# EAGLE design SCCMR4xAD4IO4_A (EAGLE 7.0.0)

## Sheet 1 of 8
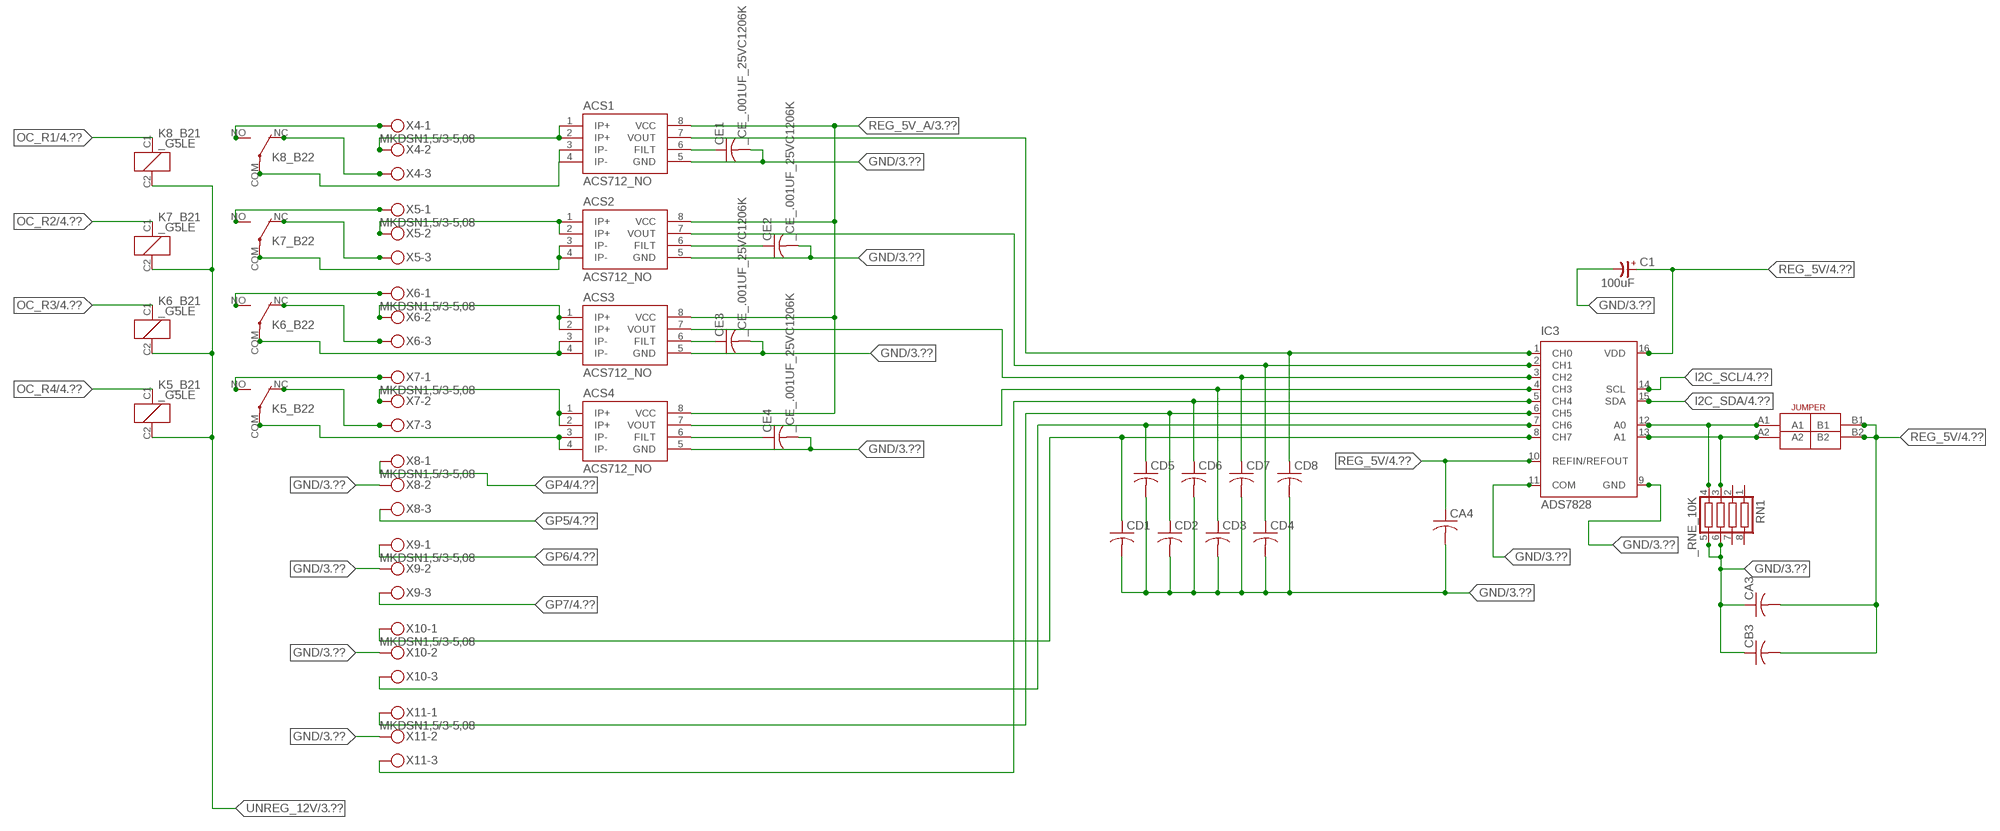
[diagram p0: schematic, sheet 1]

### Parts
ACS1  ACS712_NO  [_MA_DUAL_N-FET]
ACS2  ACS712_NO  [_MA_DUAL_N-FET]
ACS3  ACS712_NO  [_MA_DUAL_N-FET]
ACS4  ACS712_NO  [_MA_DUAL_N-FET]
C1  100uF  CP-E-025X060  [E-025X060]
CA3  CC1206KRX7R9BB104C1206K  [CC1206KRX7R9BB104]
CA4  CC1206KRX7R9BB104C1206K  [CC1206KRX7R9BB104]
CB3  TMK316F106ZL-TC1206K  [TMK316F106ZL-T]
CD1  _CD_10NF_50VC1206K  [_CD_10NF_50V]
CD2  _CD_10NF_50VC1206K  [_CD_10NF_50V]
CD3  _CD_10NF_50VC1206K  [_CD_10NF_50V]
CD4  _CD_10NF_50VC1206K  [_CD_10NF_50V]
CD5  _CD_10NF_50VC1206K  [_CD_10NF_50V]
CD6  _CD_10NF_50VC1206K  [_CD_10NF_50V]
CD7  _CD_10NF_50VC1206K  [_CD_10NF_50V]
CD8  _CD_10NF_50VC1206K  [_CD_10NF_50V]
CE1  _CE_.001UF_25VC1206K  [CE]
CE2  _CE_.001UF_25VC1206K  [CE]
CE3  _CE_.001UF_25VC1206K  [CE]
CE4  _CE_.001UF_25VC1206K  [CE]
IC3  ADS7828  [TSSOP16-PW]
K5_B2  _G5LE  [G5LE]
K6_B2  _G5LE  [G5LE]
K7_B2  _G5LE  [G5LE]
K8_B2  _G5LE  [G5LE]
RN1  _RNE_10K  [RNE]
U$4  JUMPER_2X2  [JUMPER_2X2]
X4  MKDSN1,5/3-5,08  [MKDSN1,5/3-5,08]
X5  MKDSN1,5/3-5,08  [MKDSN1,5/3-5,08]
X6  MKDSN1,5/3-5,08  [MKDSN1,5/3-5,08]
X7  MKDSN1,5/3-5,08  [MKDSN1,5/3-5,08]
X8  MKDSN1,5/3-5,08  [MKDSN1,5/3-5,08]
X9  MKDSN1,5/3-5,08  [MKDSN1,5/3-5,08]
X10  MKDSN1,5/3-5,08  [MKDSN1,5/3-5,08]
X11  MKDSN1,5/3-5,08  [MKDSN1,5/3-5,08]

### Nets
GND: ACS1.5(GND) ACS2.5(GND) ACS3.5(GND) ACS4.5(GND) C1.- CA3.1 CA4.2 CB3.1 CD1.2 CD2.2 CD3.2 CD4.2 CD5.2 CD6.2 CD7.2 CD8.2 CE1.2 CE2.2 CE3.2 CE4.2 IC3.9(GND) IC3.11(COM) RN1.5 RN1.6 X8.2 X9.2 X10.2 X11.2 ; also sheet 3,4,6,8
GP4: X8.1 ; also sheet 4
GP5: X8.3 ; also sheet 4
GP6: X9.1 ; also sheet 4
GP7: X9.3 ; also sheet 4
I2C_SCL: IC3.14(SCL) ; also sheet 4,6
I2C_SDA: IC3.15(SDA) ; also sheet 4,6
N$7: ACS1.1(IP+) ACS1.2(IP+) X4.2
N$8: CD5.1 IC3.7(CH6) X10.3
N$9: ACS1.7(VOUT) CD8.1 IC3.1(CH0)
N$10: ACS2.7(VOUT) CD4.1 IC3.2(CH1)
N$11: ACS3.7(VOUT) CD7.1 IC3.3(CH2)
N$12: ACS4.7(VOUT) CD3.1 IC3.4(CH3)
N$13: ACS2.1(IP+) ACS2.2(IP+) X5.2
N$17: IC3.12(A0) RN1.4 U$4.A1
N$18: IC3.13(A1) RN1.3 U$4.A2
N$20: CD2.1 IC3.6(CH5) X11.1
N$21: ACS4.1(IP+) ACS4.2(IP+) X7.2
N$22: ACS4.3(IP-) ACS4.4(IP-) K5_B2.COM(2:COM)
N$24: CD1.1 IC3.8(CH7) X10.1
N$25: CD6.1 IC3.5(CH4) X11.3
N$33: ACS1.6(FILT) CE1.1
N$34: ACS2.6(FILT) CE2.1
N$35: ACS3.6(FILT) CE3.1
N$36: ACS4.6(FILT) CE4.1
N$42: ACS1.3(IP-) ACS1.4(IP-) K8_B2.COM(2:COM)
N$43: K8_B2.NC(2:NC) X4.3
N$44: K8_B2.NO(2:NO) X4.1
N$45: K7_B2.NO(2:NO) X5.1
N$46: K6_B2.NO(2:NO) X6.1
N$137: K7_B2.NC(2:NC) X5.3
N$138: ACS2.3(IP-) ACS2.4(IP-) K7_B2.COM(2:COM)
N$139: K6_B2.NC(2:NC) X6.3
N$140: ACS3.3(IP-) ACS3.4(IP-) K6_B2.COM(2:COM)
N$141: K5_B2.NC(2:NC) X7.3
N$143: K5_B2.NO(2:NO) X7.1
N$166: ACS3.1(IP+) ACS3.2(IP+) X6.2
OC_R1: K8_B2.C1(1:C1) ; also sheet 4
OC_R2: K7_B2.C1(1:C1) ; also sheet 4
OC_R3: K6_B2.C1(1:C1) ; also sheet 4
OC_R4: K5_B2.C1(1:C1) ; also sheet 4
REG_5V: C1.+ CA3.2 CA4.1 CB3.2 IC3.10(REFIN/REFOUT) IC3.16(VDD) U$4.B1 U$4.B2 ; also sheet 4,6,8
REG_5V_A: ACS1.8(VCC) ACS2.8(VCC) ACS3.8(VCC) ACS4.8(VCC) ; also sheet 3
UNREG_12V: K5_B2.C2(1:C2) K6_B2.C2(1:C2) K7_B2.C2(1:C2) K8_B2.C2(1:C2) ; also sheet 3,4,6
Unconnected: RN1.1 RN1.2 RN1.7 RN1.8

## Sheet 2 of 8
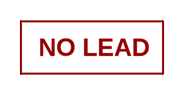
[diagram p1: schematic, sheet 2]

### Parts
U$16  NOPB_LOGO_SYM  [NOPB_LOGO_SYM]

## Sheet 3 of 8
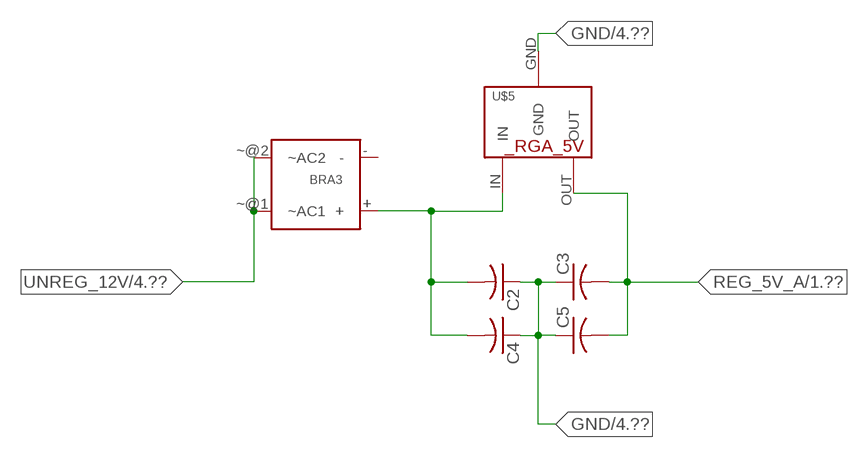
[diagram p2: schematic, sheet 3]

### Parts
BRA3  MB2S_  [MB2S]
C2  _CA_.10UF_50VC1206K  [_CA_.1UF_50V]
C3  _CA_.10UF_50VC1206K  [_CA_.1UF_50V]
C4  _CB_10UF_25VC1206K  [_CB_10UF_25V]
C5  _CB_10UF_25VC1206K  [_CB_10UF_25V]
U$5  _RGA_5V  [_RGA_5V]

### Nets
GND: C2.1 C3.1 C4.1 C5.1 U$5.GND ; also sheet 1,4,6,8
N$31: BRA3.+ C2.2 C4.2 U$5.IN
REG_5V_A: C3.2 C5.2 U$5.OUT ; also sheet 1
UNREG_12V: BRA3.~@1(~AC1) BRA3.~@2(~AC2) ; also sheet 1,4,6
Unconnected: BRA3.-

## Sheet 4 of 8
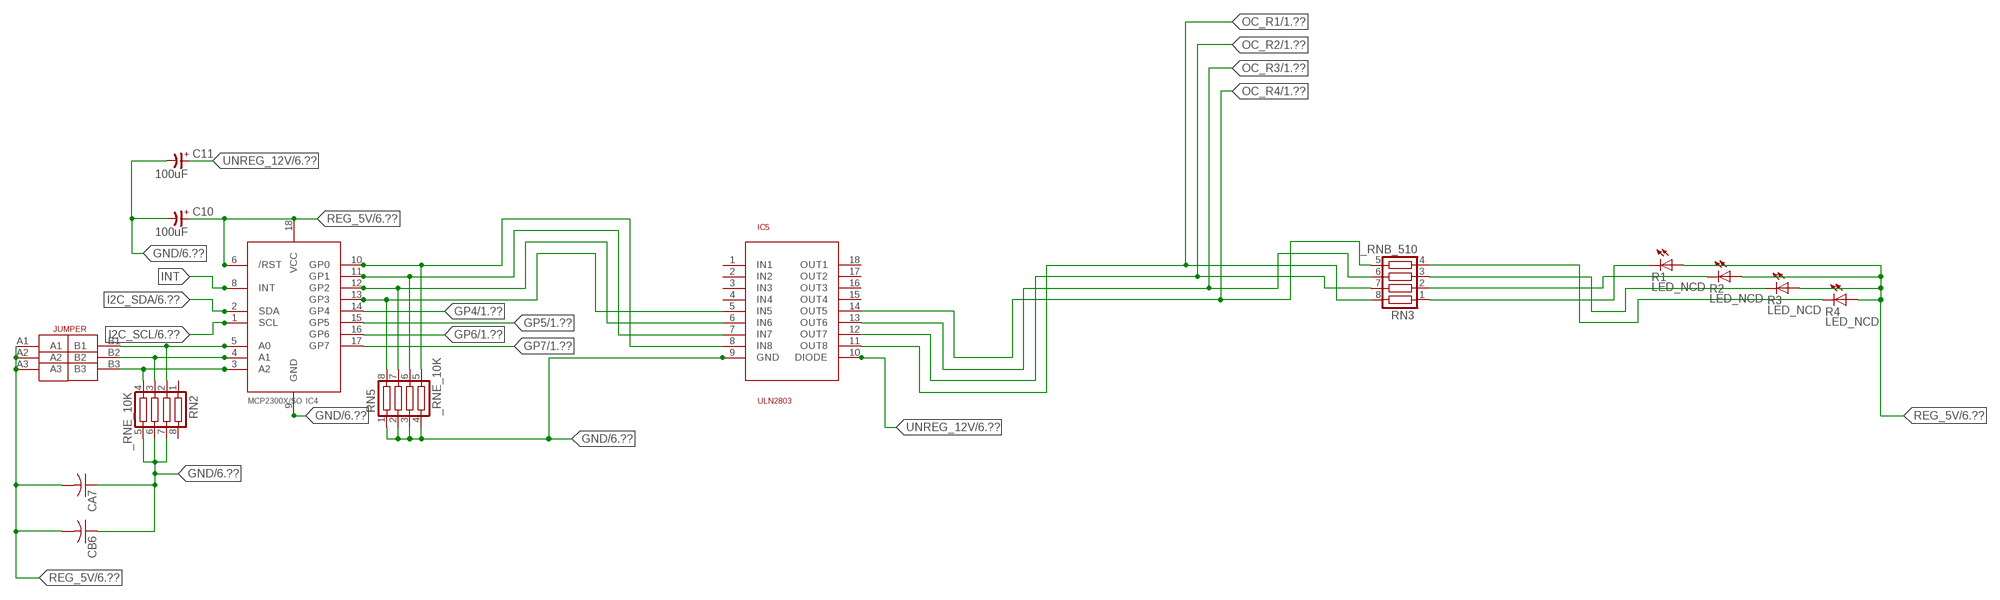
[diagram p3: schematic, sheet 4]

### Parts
C10  100uF  CP-E-025X060  [E-025X060]
C11  100uF  CP-E-025X060  [E-025X060]
CA7  CC1206KRX7R9BB104C1206K  [CC1206KRX7R9BB104]
CB6  TMK316F106ZL-TC1206K  [TMK316F106ZL-T]
IC4  MCP2300X/SO  [SO18W]
IC5  ULN2803  [SO18L]
R1  LED_NCD  [CHIPLED_0603]
R2  LED_NCD  [CHIPLED_0603]
R3  LED_NCD  [CHIPLED_0603]
R4  LED_NCD  [CHIPLED_0603]
RN2  _RNE_10K  [RNE]
RN3  _RNB_510  [RNB]
RN5  _RNE_10K  [RNE]
U$18  JUMPER_3X2  [JUMPER_3X2]

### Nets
GND: C10.- C11.- CA7.1 CB6.1 IC4.9(GND) IC5.9(GND) RN2.5 RN2.6 RN2.7 RN5.1 RN5.2 RN5.3 RN5.4 ; also sheet 1,3,6,8
GP4: IC4.14(GP4) ; also sheet 1
GP5: IC4.15(GP5) ; also sheet 1
GP6: IC4.16(GP6) ; also sheet 1
GP7: IC4.17(GP7) ; also sheet 1
I2C_SCL: IC4.1(SCL) ; also sheet 1,6
I2C_SDA: IC4.2(SDA) ; also sheet 1,6
INT: IC4.8(INT)
N$47: IC4.5(A0) RN2.2 U$18.B1
N$48: IC4.4(A1) RN2.3 U$18.B2
N$49: IC4.3(A2) RN2.4 U$18.B3
N$50: IC4.12(GP2) IC5.6(IN6) RN5.7
N$51: IC4.11(GP1) IC5.7(IN7) RN5.6
N$52: IC4.10(GP0) IC5.8(IN8) RN5.5
N$53: R1.C RN3.1
N$54: R2.C RN3.2
N$55: R3.C RN3.3
N$56: R4.C RN3.4
N$89: IC4.13(GP3) IC5.5(IN5) RN5.8
OC_R1: IC5.11(OUT8) RN3.8 ; also sheet 1
OC_R2: IC5.12(OUT7) RN3.7 ; also sheet 1
OC_R3: IC5.13(OUT6) RN3.6 ; also sheet 1
OC_R4: IC5.14(OUT5) RN3.5 ; also sheet 1
REG_5V: C10.+ CA7.2 CB6.2 IC4.6(/RST) IC4.18(VCC) R1.A R2.A R3.A R4.A U$18.A1 U$18.A2 U$18.A3 ; also sheet 1,6,8
UNREG_12V: C11.+ IC5.10(DIODE) ; also sheet 1,3,6
Unconnected: IC5.1(IN1) IC5.2(IN2) IC5.3(IN3) IC5.4(IN4) IC5.15(OUT4) IC5.16(OUT3) IC5.17(OUT2) IC5.18(OUT1) RN2.1 RN2.8

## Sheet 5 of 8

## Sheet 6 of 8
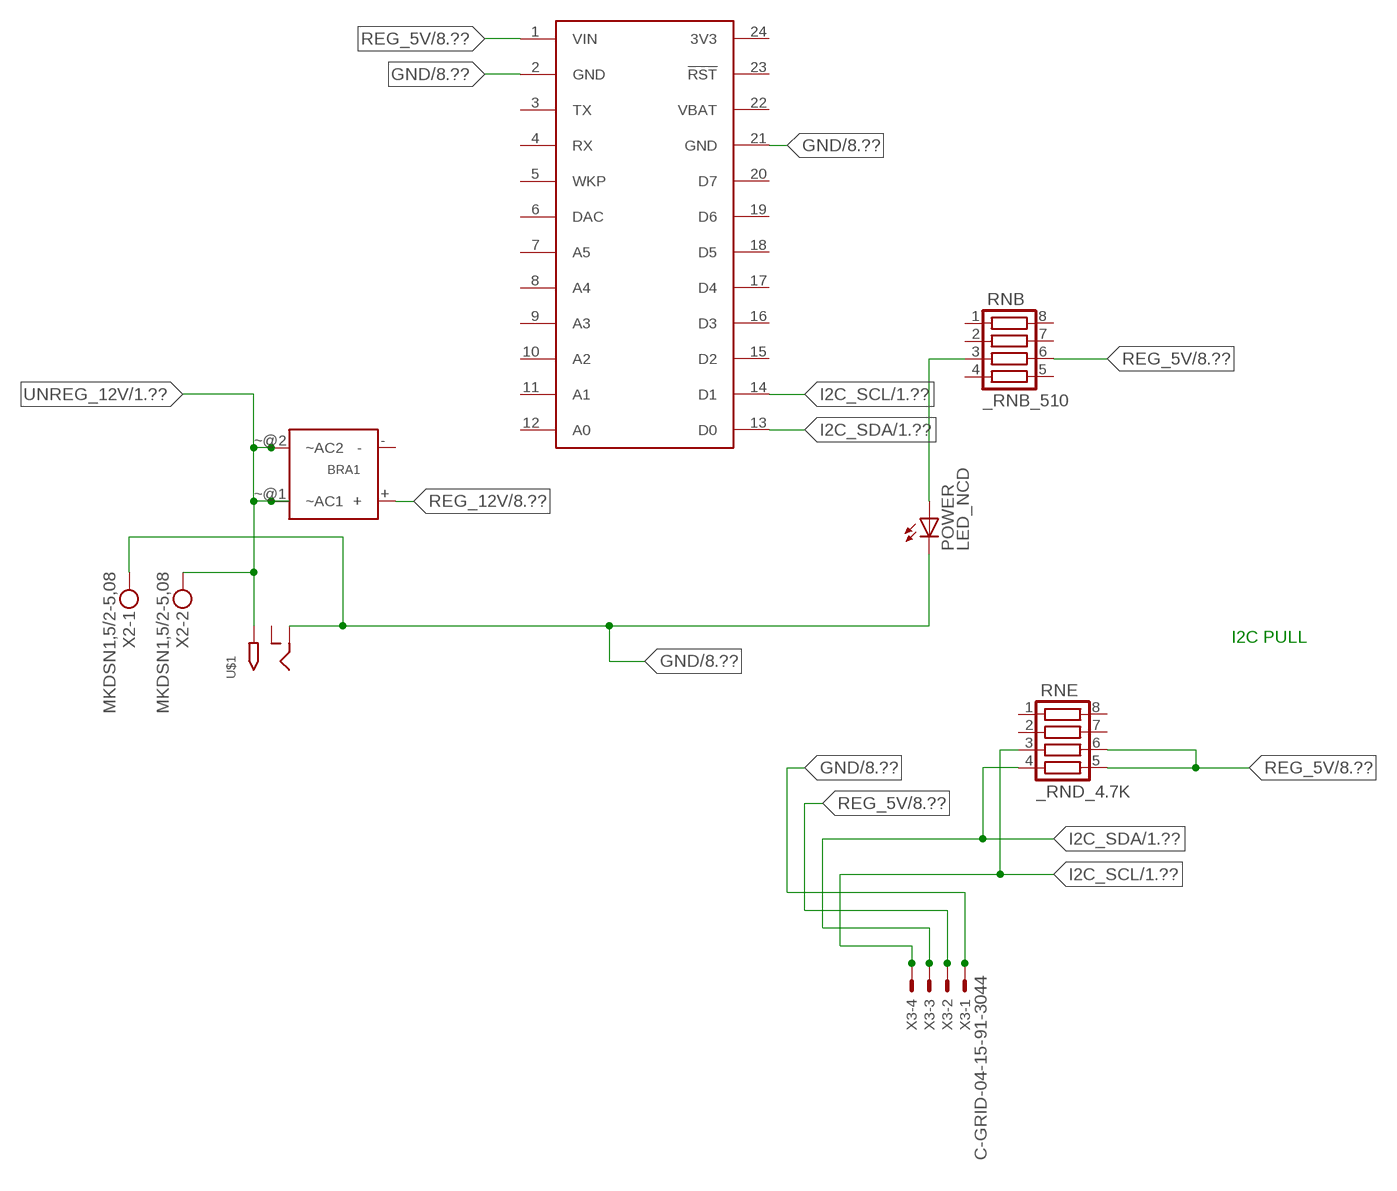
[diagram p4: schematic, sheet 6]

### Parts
BRA1  MB2S_  [MB2S]
POWER  LED_NCD  [CHIPLED_0603]
RNB  _RNB_510  [RNB]
RNE  _RND_4.7K  [RND]
S1  SPARK_CORECORE  [SPARK_CORE]
U$1  2.1MMJACK  [PJ-102A]
X2  MKDSN1,5/2-5,08  [MKDSN1,5/2-5,08]
X3  C-GRID-04-15-91-3044  [15-91-04]

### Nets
GND: POWER.C S1.2(GND) S1.21(GND) U$1.RING X2.1 X3.1 ; also sheet 1,3,4,8
I2C_SCL: RNE.3 S1.14(D1) X3.4 ; also sheet 1,4
I2C_SDA: RNE.4 S1.13(D0) X3.3 ; also sheet 1,4
N$2: POWER.A RNB.3
REG_5V: RNB.6 RNE.5 RNE.6 S1.1(VIN) X3.2 ; also sheet 1,4,8
REG_12V: BRA1.+ ; also sheet 8
UNREG_12V: BRA1.~@1(~AC1) BRA1.~@2(~AC2) U$1.TIP X2.2 ; also sheet 1,3,4
Unconnected: BRA1.- RNB.1 RNB.2 RNB.4 RNB.5 RNB.7 RNB.8 RNE.1 RNE.2 RNE.7 RNE.8 S1.3(TX) S1.4(RX) S1.5(WKP) S1.6(DAC) S1.7(A5) S1.8(A4) S1.9(A3) S1.10(A2) S1.11(A1) S1.12(A0) S1.15(D2) S1.16(D3) S1.17(D4) S1.18(D5) S1.19(D6) S1.20(D7) S1.23(!RST) U$1.RING_SW

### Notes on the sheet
- I2C PULL

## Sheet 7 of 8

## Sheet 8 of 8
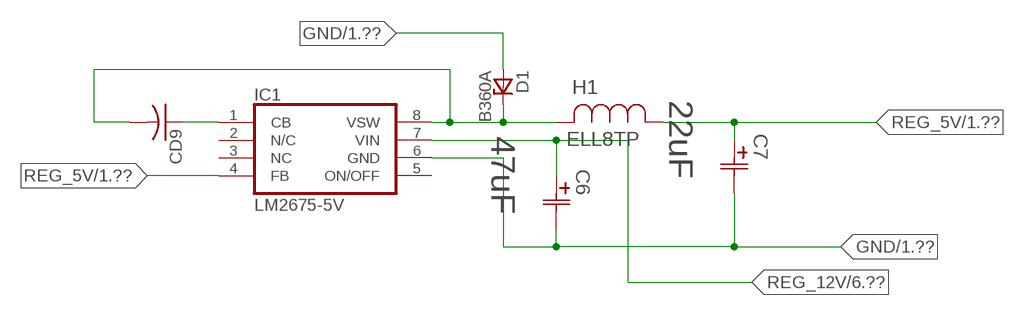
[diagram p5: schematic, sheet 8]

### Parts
C6  47uF  490-5463-6-NDCAP  [C2917(7343)-Y]
C7  22uF  490-5463-6-NDCAP  [C2917(7343)-Y]
CD9  _CD_10NF_50VC1206K  [_CD_10NF_50V]
D1  B360A  [DO214AC_ZENER]
H1  ELL8TP  [IND_ELL8TP]
IC1  LM2675-5V  LM2675  [SO-8]

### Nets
GND: C6.2(C2) C7.2(C2) D1.A IC1.6(GND) ; also sheet 1,3,4,6
N$1: CD9.2 D1.C H1.2 IC1.8(VSW)
N$6: CD9.1 IC1.1(CB)
REG_5V: C7.1(C1) H1.1 IC1.4(FB) ; also sheet 1,4,6
REG_12V: C6.1(C1) IC1.7(VIN) ; also sheet 6
Unconnected: IC1.2(N/C) IC1.5(ON/OFF)

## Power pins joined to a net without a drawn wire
3V3: S1.24(3V3)
NC: IC1.3(NC)
VBAT: S1.22(VBAT)

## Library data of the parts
ACS1-ACS4 = NCD_ULTIMATE_LIBRARY:ACS712_NO: Semiconductor Sensor Current Hall-effect-based isolated linear current sensor Digikey 620-1190-2-ND/ACS712ELCTR-20A-T
BRA1 BRA3 = NCD_ULTIMATE_LIBRARY:MB2S: Bridge Rectifier BRA MB2S 200V 500ma Digikey MB2S-TPMSTR-ND/MB2S-TP
C1 C10 C11 = NCD_ULTIMATE_LIBRARY:CP-: Capacitors All Kinds POLARIZED CAP
C2 C3 = NCD_ULTIMATE_LIBRARY:_CA_.10UF_50V: Capacitor .1uF SMT
C4 C5 = NCD_ULTIMATE_LIBRARY:_CB_10UF_25V: Capacitor 10uF SMT
C6 C7 = NCD_ULTIMATE_bhaskar:490-5463-6-ND: NCD CAP
CA3 CA4 CA7 = NCD_ULTIMATE_LIBRARY:CC1206KRX7R9BB104: Capacitor CA .1uF 50V SMT C1206K CC1206KRX7R9BB104
CB3 CB6 = NCD_ULTIMATE_LIBRARY:TMK316F106ZL-T: Capacitor CB 10uF SMT 1206 TMK316F106ZL-T
CD1-CD9 = NCD_ULTIMATE_LIBRARY:_CD_10NF_50V: Capacitor 10nF SMT
CE1-CE4 = NCD_ULTIMATE_LIBRARY:_CE_.001UF_25V: Capacitor .001uF SMT
D1 = NCD_ULTIMATE_bhaskar:B360A: NCD DIODE B350A/B360A
H1 = NCD_ULTIMATE_bhaskar:ELL8TP: NCD coil
IC1 = NCD_ULTIMATE_bhaskar:LM2675: LM2675 NCD http://www.ti.com/lit/ds/symlink/lm2675.pdf
IC3 = NCD_ULTIMATE_LIBRARY:ADS7828: Semiconductor ADC I2C 12-Bit, 8-Channel Sampling ANALOG-TO-DIGITAL CONVERTER Digikey 296-12402-2-ND Source: www.ti.com .. ADS7828.pdf / ADS7828E/250; MF: TEXAS INSTRUMENTS; MPN: ADS7828E/250; OC_FARNELL: 1470338; OC_NEWARK: 74C7158
IC4 = NCD_ULTIMATE_LIBRARY:MCP2300X: Semiconductor Port Expander I/O 8-Bit I2C MCP23008 Inexpensive i2c i/o expander - 8 general purpose i/o pins with optional pullups
IC5 = NCD_ULTIMATE_LIBRARY:ULN2803: Semiconductor 8 O.C. N-Channel Transistor Driver Digikey ULN2803AFWGCELTR-ND/ULN2803AFWG,C,EL
K5_B2 K6_B2 K7_B2 K8_B2 = NCD_ULTIMATE_LIBRARY:_G5LE: Relay 5A/10A SPDT; OC_FARNELL: unknown; OC_NEWARK: unknown
POWER = NCD_ULTIMATE_bhaskar:LED_NCD
R1-R4 = NCD_ULTIMATE_LIBRARY:LED_NCD: LED Digikey 754-1132-2-ND/APT2012SRCPRV
RN1 RN2 RN5 = NCD_ULTIMATE_LIBRARY:_RNE_10K: Resistor Array RNE SMT 10K x 4 Single Resistor Source: http://www.ctscorp.com/components/Datasheets/CTSChipArrayDs.pdf Digikey 742C083103JPTR-ND/742C083103JP; OC_FARNELL: unknown; OC_NEWARK: unknown
RN3 RNB = NCD_ULTIMATE_LIBRARY:_RNB_510: Resistor Array RNB SMT 510 x 4 Single Resistor Source: http://www.ctscorp.com/components/Datasheets/CTSChipArrayDs.pdf Digikey 742C083511JPTR-ND/ 742C083511JP; OC_FARNELL: unknown; OC_NEWARK: unknown
RNE = NCD_ULTIMATE_LIBRARY:_RND_4.7K: Resistor Array RND SMT 4.7K x 4 Single Resistor Source: http://www.ctscorp.com/components/Datasheets/CTSChipArrayDs.pdf Digikey 742C083472JPTR-ND/742C083472JP; OC_FARNELL: unknown; OC_NEWARK: unknown
S1 = Spark:SPARK_CORE
U$1 = NCD_ULTIMATE_CONNECTORS:2.1MMJACK: 2.1mm x 5.5mm DC jack with internal switch. Digikey part #PJ-102A, 4UCON part #05537 By microbuilder.eu
U$4 = NCD_ULTIMATE_CONNECTORS:JUMPER_2X2
U$5 = NCD_ULTIMATE_LIBRARY:_RGA_5V: Regulator Linear 5V Digikey 497-7255-2-ND/ L7805CDT-TR
U$16 = PatternAgents-Logos:NOPB_LOGO_SYM: NOPB_LOGO_SYM
U$18 = NCD_ULTIMATE_CONNECTORS:JUMPER_3X2
X2 = NCD_ULTIMATE_CONNECTORS:MKDSN1,5/2-5,08: MKDSN 1,5/ 2-5,08 Printklemme
X3 = NCD_ULTIMATE_CONNECTORS:C-GRID-04: CONNECTOR 4-Pos I2C wire to board 2.54 mm (0.100") pitch header Digikey WM1342-ND/0015912045; OC_FARNELL: unknown; OC_NEWARK: unknown
X4-X11 = NCD_ULTIMATE_CONNECTORS:MKDSN1,5/3-5,08: MKDSN 1,5/ 3-5,08 Printklemme Nennstrom: 13,5 A Nennspannung: 250 V Rastermaß: 5,08 mm Polzahl: 3 Anschlussart: Schraubanschluss Montage: Löten Anschlussrichtung Leiter/Platine: 0 ° Artikelnummer: 1729131 Source: http://eshop.phoenixcontact.com .. 1729131.pdf

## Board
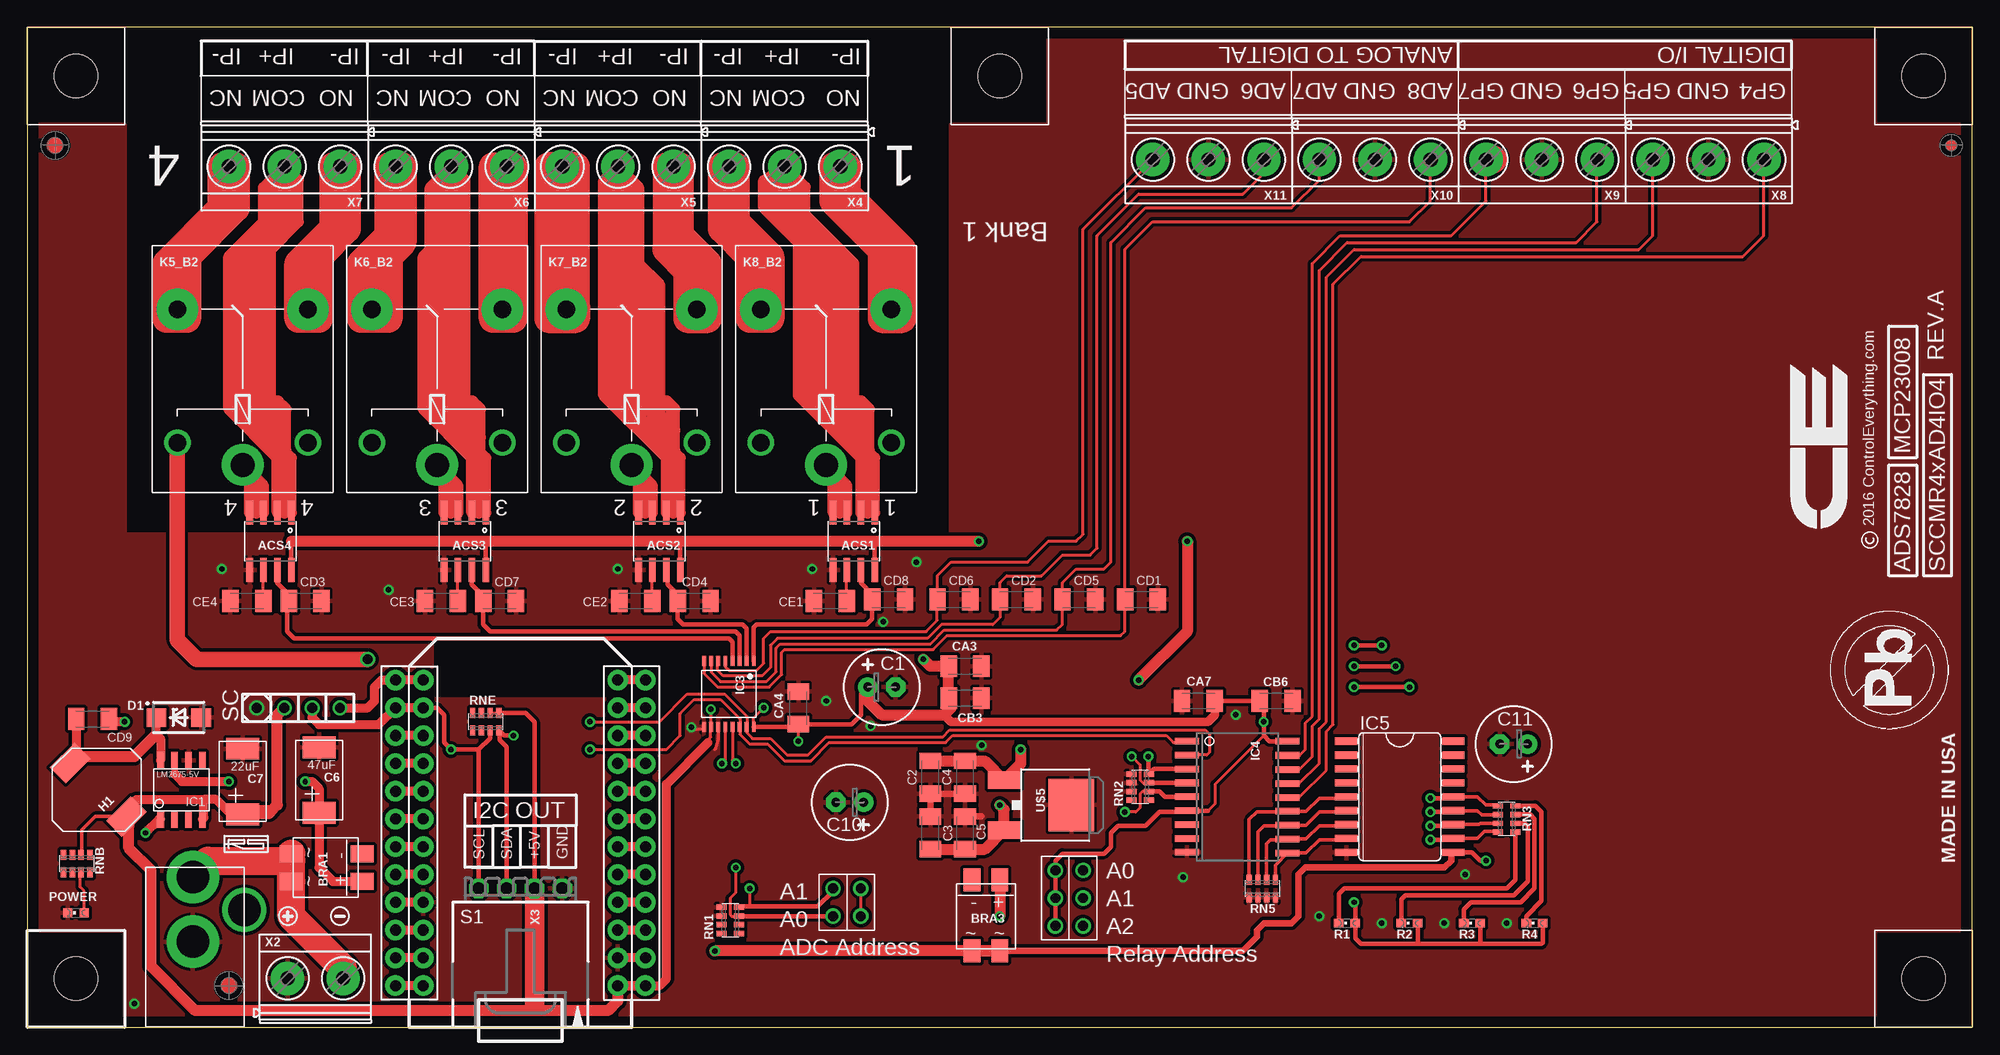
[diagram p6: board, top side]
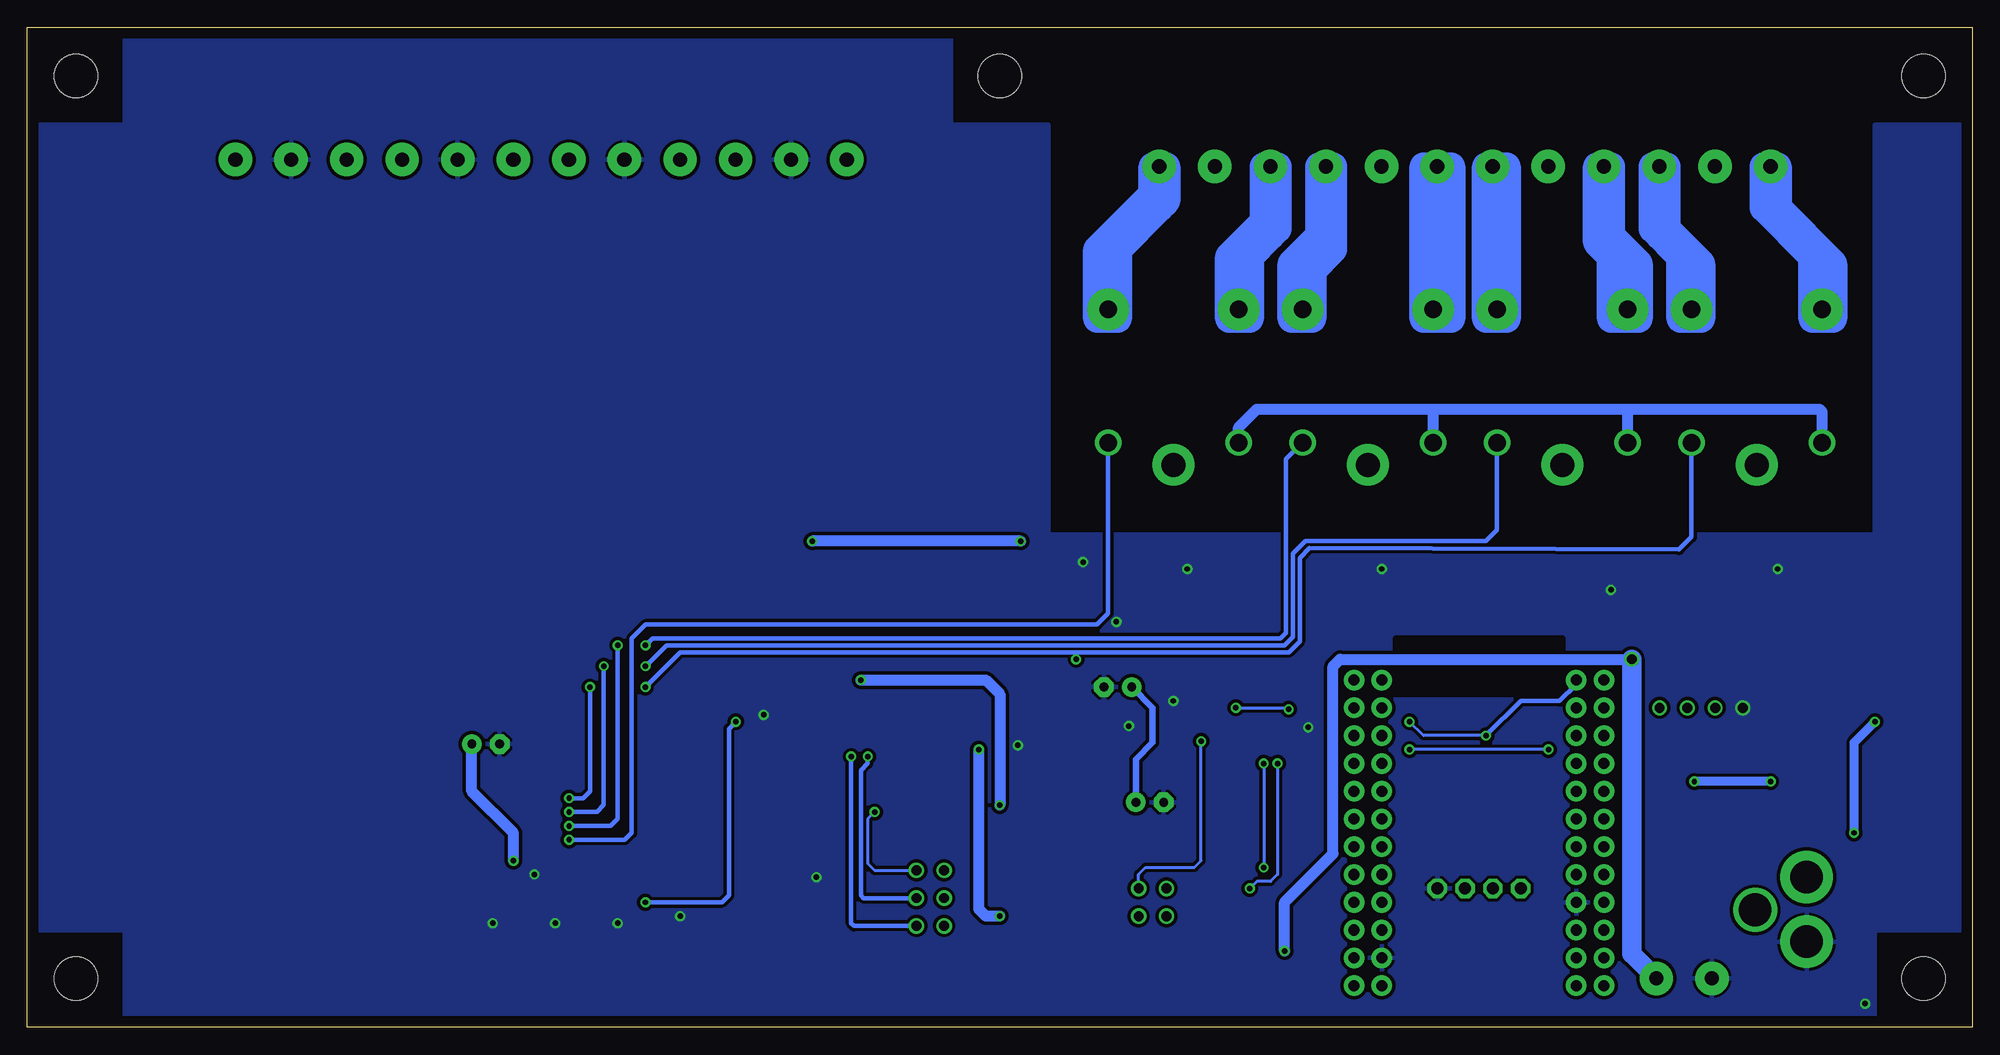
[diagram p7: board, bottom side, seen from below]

Size 177.8 x 91.44 mm. Coordinates in mm from the lower left corner, seen from the top.
Outline: 0,91.11 0,90.17
Outline: 0,90.17 0,0 177.8,0 177.8,91.44 0,91.44 0,90.17
Copper layers (1*16): Top 0.035mm / dielectric 1.5mm / Bottom 0.035mm
Design rules "default": minimum track width 10mil, minimum drill 24mil, track to track 8mil, track to pad 8mil, pad to pad 8mil, via to via 8mil, smd to smd 8mil, copper to edge 40mil, drill to drill 8mil, minimum pad ring 10mil, minimum via ring 8mil, stop-mask expansion 4mil, vias tented up to drill 0mil, thermal gap 10mil
Holes 3.96 mm at 4.45,4.45 4.45,4.45

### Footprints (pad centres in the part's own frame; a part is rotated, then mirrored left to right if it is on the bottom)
_MA_DUAL_N-FET = smd 0.61 x 2.21: 1 -1.905,-2.616; 2 -0.635,-2.616; 3 0.635,-2.616; 4 1.905,-2.616; 5 1.905,2.616; 6 0.635,2.616; 7 -0.635,2.616; 8 -1.905,2.616
MB2S = smd 1.55 x 2.1: + 0,-6.5; - 2.54,-6.5; ~@1 0,0; ~@2 2.54,0
E-025X060 = drill 0.813 pad 1.778: + -1.27,0 | drill 0.813 pad 1.778 octagon: - 1.27,0
_CA_.1UF_50V = smd 1.5 x 2: 1 -1.5,0; 2 1.5,0
_CB_10UF_25V = smd 1.5 x 2: 1 -1.5,0; 2 1.5,0
C2917(7343)-Y = smd 2 x 3: 1 -3,0; 2 3,0
CC1206KRX7R9BB104 = smd 1.5 x 2: 1 -1.5,0; 2 1.5,0
TMK316F106ZL-T = smd 1.5 x 2: 1 -1.5,0; 2 1.5,0
_CD_10NF_50V = smd 1.5 x 2: 1 -1.5,0; 2 1.5,0
CE = smd 1.5 x 2: 1 -1.5,0; 2 1.5,0
DO214AC_ZENER = smd 1.8 x 1.7: A 2.05,0; C -2.05,0
IND_ELL8TP = smd 2.054 x 3.2 rotated 45: 1 -2.442,-2.696; 2 2.442,2.442
SO-8 = smd 0.6 x 1.55: 1 -1.905,-2.69; 2 -0.635,-2.69; 3 0.635,-2.69; 4 1.905,-2.69; 5 1.905,2.71; 6 0.635,2.71; 7 -0.635,2.71; 8 -1.905,2.71
TSSOP16-PW = smd 0.35 x 0.9: 1 -2.275,-3.025; 2 -1.625,-3.025; 3 -0.975,-3.025; 4 -0.325,-3.025; 5 0.325,-3.025; 6 0.975,-3.025; 7 1.625,-3.025; 8 2.275,-3.025; 9 2.275,3.025; 10 1.625,3.025; 11 0.975,3.025; 12 0.325,3.025; 13 -0.325,3.025; 14 -0.975,3.025; 15 -1.625,3.025; 16 -2.275,3.025
SO18W = smd 0.6 x 2.2: 1 -4.445,-4.6; 2 -3.175,-4.6; 3 -1.905,-4.6; 4 -0.635,-4.6; 5 0.635,-4.6; 6 1.905,-4.6; 7 3.175,-4.6; 8 4.445,-4.6; 9 5.715,-4.6; 10 5.775,4.6; 11 4.505,4.6; 12 3.235,4.6; 13 1.965,4.6; 14 0.695,4.6; 15 -0.575,4.6; 16 -1.845,4.6; 17 -3.145,4.6; 18 -4.445,4.6
SO18L = smd 0.66 x 2.032: 1 -5.08,-4.902; 2 -3.81,-4.902; 3 -2.54,-4.902; 4 -1.27,-4.902; 5 0,-4.902; 6 1.27,-4.902; 7 2.54,-4.902; 8 3.81,-4.902; 9 5.08,-4.902; 10 5.08,4.902; 11 3.81,4.902; 12 2.54,4.902; 13 1.27,4.902; 14 0,4.902; 15 -1.27,4.902; 16 -2.54,4.902; 17 -3.81,4.902; 18 -5.08,4.902
G5LE = drill 1.6: C1 -7.493,-5.969; C2 -7.493,5.969 | drill 2.2 pad 3.81: COM -9.525,0 | drill 1.6 pad 3.81: NC 4.699,5.969; NO 4.699,-5.969
CHIPLED_0603 = smd 0.8 x 0.8: A 0,-0.75; C 0,0.75
CHIPLED_0603' = smd 0.8 x 0.876: A 0,-0.75; C 0,0.75
RNE = smd 0.5 x 0.9: 1 -1.2,-0.8; 2 -0.4,-0.8; 3 0.4,-0.8; 4 1.2,-0.8; 5 1.2,0.8; 6 0.4,0.8; 7 -0.4,0.8; 8 -1.2,0.8
RNB = smd 0.5 x 0.9: 1 -1.2,-0.8; 2 -0.4,-0.8; 3 0.4,-0.8; 4 1.2,-0.8; 5 1.2,0.8; 6 0.4,0.8; 7 -0.4,0.8; 8 -1.2,0.8
RND = smd 0.5 x 0.9: 1 -1.2,-0.8; 2 -0.4,-0.8; 3 0.4,-0.8; 4 1.2,-0.8; 5 1.2,0.8; 6 0.4,0.8; 7 -0.4,0.8; 8 -1.2,0.8
SPARK_CORE = drill 1.016 pad 1.88: 1 -8.89,13.97; 2 -8.89,11.43; 3 -8.89,8.89; 4 -8.89,6.35; 5 -8.89,3.81; 6 -8.89,1.27; 7 -8.89,-1.27; 8 -8.89,-3.81; 9 -8.89,-6.35; 10 -8.89,-8.89; 11 -8.89,-11.43; 12 -8.89,-13.97; 13 8.89,-13.97; 14 8.89,-11.43; 15 8.89,-8.89; 16 8.89,-6.35; 17 8.89,-3.81; 18 8.89,-1.27; 19 8.89,1.27; 20 8.89,3.81; 21 8.89,6.35; 22 8.89,8.89; 23 8.89,11.43; 24 8.89,13.97; 25 -11.43,13.97; 26 -11.43,11.43; 27 -11.43,8.89; 28 -11.43,6.35; 29 -11.43,3.81; 30 -11.43,1.27; 31 -11.43,-1.27; 32 -11.43,-3.81; 33 -11.43,-6.35; 34 -11.43,-8.89; 35 -11.43,-11.43; 36 -11.43,-13.97; 37 11.43,13.97; 38 11.43,11.43; 39 11.43,8.89; 40 11.43,6.35; 41 11.43,3.81; 42 11.43,1.27; 43 11.43,-1.27; 44 11.43,-3.81; 45 11.43,-6.35; 46 11.43,-8.89; 47 11.43,-11.43; 48 11.43,-13.97
PJ-102A = drill 3 pad 4.8: RING 0.1,-3.39; TIP 0.1,-9.29 | drill 3 pad 3.251: RING_SW -4.6,-6.29
JUMPER_2X2 = drill 0.9: A1 0,2.54; A2 0,0; B1 2.54,2.54; B2 2.54,0
_RGA_5V = smd 4.826 x 4.191: GND 0,2.096 | smd 1.6 x 3: IN -2.28,-4.04; OUT 2.28,-4.04
PCB_MOUNTING_HOLE = hole 3.962: 4.445,4.445
JUMPER_3X2 = drill 0.9: A1 0,5.08; A2 0,2.54; A3 0,0; B1 2.54,5.08; B2 2.54,2.54; B3 2.54,0
MKDSN1,5/2-5,08 = drill 1.3 pad 3.048: 1 -2.561,0.025; 2 2.519,0.025
15-91-04 = drill 1.1 pad 1.778 octagon: 1 -3.81,-7.62; 2 -1.27,-7.62; 3 1.27,-7.62; 4 3.81,-7.62
MKDSN1,5/3-5,08 = drill 1.3 pad 3.048: 1 -7.641,0.025; 2 -2.561,0.025; 3 2.519,0.025

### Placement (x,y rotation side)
ACS1  75.56,44.45 180 top
ACS2  57.78,44.45 180 top
ACS3  40.01,44.45 180 top
ACS4  22.23,44.45 180 top
BRA1  24.13,13.34 90 top
BRA3  88.9,6.99 180 top
C1  78.11,31.12 0 top
C2  82.55,22.86 90 top
C3  82.55,17.78 270 top
C4  85.72,22.86 90 top
C5  85.72,17.78 270 top
C6  26.67,22.61 90 top
C7  19.68,22.48 90 top
C10  75.18,20.57 180 top
C11  135.89,25.91 180 top
CA3  85.72,33.02 180 top
CA4  70.48,29.21 90 top
CA7  107.06,29.84 0 top
CB3  85.72,30.1 180 top
CB6  114.17,29.84 180 top
CD1  101.85,39.12 0 top
CD2  90.42,39.12 0 top
CD3  25.4,38.99 0 top
CD4  60.96,38.99 0 top
CD5  96.14,39.12 0 top
CD6  84.71,39.12 0 top
CD7  43.18,38.99 0 top
CD8  78.74,39.12 0 top
CD9  5.97,28.19 180 top
CE1  73.41,38.99 180 top
CE2  55.63,38.99 180 top
CE3  37.85,38.99 180 top
CE4  20.07,38.99 180 top
D1  13.84,28.32 0 top
H1  6.35,21.72 90 top
IC1  14.1,21.72 0 top
IC3  64.14,30.48 180 top
IC4  110.62,21.72 270 top
IC5  125.48,21.08 270 top
K5_B2  19.68,60.96 90 top
K6_B2  37.47,60.96 90 top
K7_B2  55.24,60.96 90 top
K8_B2  73.03,60.96 90 top
POWER  4.45,10.48 90 top
R1  LED_NCD  [CHIPLED_0603']  120.65,9.53 90 top
R2  LED_NCD  [CHIPLED_0603']  126.36,9.53 90 top
R3  LED_NCD  [CHIPLED_0603']  132.08,9.53 90 top
R4  LED_NCD  [CHIPLED_0603']  137.79,9.53 90 top
RN1  64.26,9.78 90 top
RN2  101.73,21.97 90 top
RN3  135.25,19.05 90 top
RN5  112.9,12.7 0 top
RNB  4.51,14.99 0 top
RNE  41.91,27.94 0 top
S1  45.09,17.78 180 top
U$1  15.24,4.45 180 top
U$4  73.66,10.16 0 top
U$5  93.34,20.32 270 top
U$10  [VISION_REF15]  18.41,3.81 0 top
U$15  PCB_MOUNTING_HOLE  [PCB_MOUNTING_HOLE]  177.8,0 90 top
U$16  176.07,27.08 90 top
U$18  93.98,9.27 0 top
U$20  PCB_MOUNTING_HOLE  [PCB_MOUNTING_HOLE]  177.8,82.55 90 top
U$21  [ICON_USA]  175.01,26.92 270 top
U$22  [ICON_MINUS]  28.57,10.16 180 top
U$23  PCB_MOUNTING_HOLE  [PCB_MOUNTING_HOLE]  93.34,82.55 90 top
U$24  [ICON_PLUS]  23.81,10.16 90 top
U$25  PCB_MOUNTING_HOLE  [PCB_MOUNTING_HOLE]  8.89,82.55 90 top
U$26  PCB_MOUNTING_HOLE  [PCB_MOUNTING_HOLE]  177.8,82.55 90 top
U$27  [VISION_REF15]  2.54,80.65 270 top
U$28  [VISION_REF10]  175.9,80.65 270 top
X2  26.35,4.45 0 top
X3  45.09,5.08 180 top
X4  66.67,78.74 180 top
X5  51.44,78.74 180 top
X6  36.2,78.74 180 top
X7  20.95,78.74 180 top
X8  151.13,79.38 180 top
X9  135.89,79.38 180 top
X10  120.65,79.38 180 top
X11  105.41,79.38 180 top

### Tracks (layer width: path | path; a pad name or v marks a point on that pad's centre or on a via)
GND  (via drill 0.5, 0.9)
  Top 0.254: 62.87,25.4 63.16,26.33 IC3.11 63.16,26.46 63.12,26.42 | 60.96,27.3 61.71,27.3 IC3.9
  Top 0.61: C4.1 C2.1 C3.1 | C5.1 87.22,19.28
  other vias: 71.75,41.91 73.03,29.84 53.98,41.91 33.02,40.01 105.66,13.72 118.11,10.16 135.25,9.53 129.54,9.53 123.83,9.53 110.49,28.57 77.09,27.56 87.25,25.78 131.44,13.97 17.78,41.91 81.28,42.55 78.23,37.08 9.78,2.16 20.95,29.21 60.71,27.43
  pour Top (isolate 0.305): 8.89,-1.9 8.89,8.89 -2.54,8.89 -2.54,82.55 8.89,82.55 8.89,45.09 84.45,45.09 84.45,82.55 93.34,82.55 93.34,104.14 168.91,104.14 168.91,82.55 179.07,82.55 179.71,83.19 179.71,8.89 168.91,8.89 168.91,-1.27 168.28,-1.9
  pour Bottom (isolate 0.305): 8.89,-1.9 8.89,8.89 -10.16,8.89 -10.16,82.55 8.89,82.55 8.89,45.09 84.45,45.09 84.45,82.55 93.34,82.55 93.34,102.24 168.91,102.24 168.91,82.55 179.07,82.55 179.71,83.19 179.71,8.89 168.91,8.89 168.91,-1.27 168.28,-1.9
GP4
  Top 0.254: IC4.14 116.27,21.02 118.75,23.5 118.75,27.05 119.38,27.69 119.38,67.94 121.92,70.49 156.84,70.49 158.75,72.39 158.75,79.33 X8.1
GP5
  Top 0.254: IC4.15 116.27,22.29 118.11,24.13 118.11,27.3 118.75,27.94 118.75,68.58 121.28,71.12 147.32,71.12 148.59,72.39 148.59,79.33 X8.3
GP6
  Top 0.254: IC4.16 116.27,23.56 117.47,24.77 117.47,27.56 118.11,28.19 118.11,69.22 120.65,71.75 141.6,71.75 143.51,73.66 143.51,79.33 X9.1
GP7
  Top 0.254: IC4.17 116.3,24.86 116.84,25.4 116.84,27.81 117.47,28.45 117.47,69.85 120.02,72.39 130.18,72.39 133.35,75.56 133.35,79.33 X9.3
I2C_SCL  (via drill 0.5, 0.9)
  Top 0.254: 65.15,27.5 65.15,28.19 63.37,29.97 60.96,29.97 59.69,28.7 59.69,26.67 58.42,25.4 v51.44,25.4 | 65.15,27.5 IC3.14 | 65.15,27.5 65.15,26.8 66.04,25.91 67.69,25.91 69.22,24.38 71.63,24.38 73.28,26.04 83.95,26.04 84.58,26.67 104.14,26.67 104.78,26.04 105.89,26.04 IC4.1
  Top 0.406: X3.4 41.27,25.4 | 41.27,25.4 42.29,26.42 42.29,27.12 RNE.3 | S1.14 37.47,29.21 38.1,28.57 38.1,26.04 v38.73,25.4 41.27,25.4
  Top 0.813: v26.04,29.21 26.04,28.32 26.67,27.69 32.13,27.69 33.66,29.21
  Bottom 0.254: v38.73,25.4 v51.44,25.4
I2C_SDA  (via drill 0.5, 0.9)
  Top 0.254: 65.79,27.48 65.79,28.45 63.75,30.48 60.33,30.48 57.78,27.94 v51.44,27.94 | 65.79,27.48 IC3.15 | 65.79,27.48 65.79,26.92 66.29,26.42 67.94,26.42 69.47,24.89 71.37,24.89 73.03,26.54 83.69,26.54 84.33,27.18 107.7,27.18 108.08,26.8 108.08,25.15 107.82,24.89 IC4.2
  Top 0.406: X3.3 43.81,25.65 43.18,26.29 43.18,27.07 RNE.4 43.58,26.67 v44.45,26.67
  Top 0.813: v28.57,29.21 31.11,29.21 31.75,29.84 31.75,31.12 32.38,31.75 33.66,31.75
  Bottom 0.254: v44.45,26.67 50.16,26.67 v51.44,27.94
  Bottom 0.406: S1.13 36.2,31.37 37.72,29.84 41.27,29.84 v44.45,26.67
N$1
  Top 0.813: H1.2 3.88,24.77 | D1.C 11.79,26.78 12.19,26.38 IC1.8 | CD9.2 4.47,24.79 4.45,24.77
  Top 1.016: 3.88,24.77 4.45,24.77 9.78,24.77 11.79,26.78
N$2
  Top 0.254: POWER.A 5.2,12.46 4.83,12.83 4.83,14.1 RNB.3
  Top 0.406: 4.95,14.14 RNB.3
N$6  (via drill 0.5)
  Top 0.813: IC1.1 12.04,19.03 v10.79,17.78 | v8.89,27.94 7.72,27.94 CD9.1
  Bottom 0.813: v10.79,17.78 10.79,26.04 v8.89,27.94
N$7
  Top 1.016: ACS1.1 77.47,52.07 76.83,52.7 75.56,53.98 75.56,69.85 71.12,74.29 71.12,76.83 X4.2 67.31,77.42 67.31,74.93 70.48,71.75 70.48,57.79 76.2,52.07 ACS1.2
  Top 1.27: 76.83,52.7 76.83,56.52 76.2,57.15 76.2,53.98
  Top 1.778: 69.22,78.69 X4.2
N$8
  Top 0.254: IC3.7 62.51,32.49 63.37,31.62 67.56,31.62 68.45,32.51 68.45,34.67 68.83,35.05 82.55,35.05 83.82,36.32 94.11,36.32 94.61,36.83 94.61,39.09 CD5.1 94.64,40.66 95.89,41.91 98.42,41.91 99.06,42.55 99.06,71.75 102.23,74.93 115.57,74.93 118.11,77.47 118.11,79.33 X10.3
N$9
  Top 0.406: 77.47,38.89 CD8.1 | CD8.1 77.24,39.6 76.2,40.64 ACS1.7 | IC3.1 66.41,36.56 66.67,36.83 76.71,36.83 77.22,37.34 77.22,39.09 CD8.1
N$10
  Top 0.406: ACS2.7 58.55,41.71 58.55,40.51 59.46,39.6 CD4.1 59.44,38.97 59.44,37.34 59.94,36.83 65.41,36.83 65.76,36.48 IC3.2
N$11
  Top 0.406: ACS3.7 40.64,40.51 41.68,39.47 CD7.1 41.66,38.97 41.66,36.83 42.29,36.2 64.77,36.2 65.11,35.86 IC3.3
N$12
  Top 0.406: IC3.4 64.46,35.23 64.14,35.56 24.38,35.56 23.75,36.2 23.75,38.84 CD3.1 23.9,39.6 22.86,40.64 ACS4.7
N$13
  Top 1.016: ACS2.2 58.42,52.07 52.7,57.79 52.7,77.42 X5.2 55.24,77.47 55.25,77.47 55.88,76.84 55.88,69.85 57.78,67.94 57.78,57.15 57.78,55.88 57.78,53.98 59.05,52.7 59.69,52.07 ACS2.1
  Top 1.27: 59.05,52.7 59.05,54.61 | 59.05,54.61 57.78,55.88 57.78,54.61 58.42,53.98 | 59.05,54.61 59.05,56.52 58.42,57.15 57.78,57.15
N$17  (via drill 0.5)
  Top 0.254: IC3.12 63.81,24.44 v63.5,24.13 | v66.04,12.7 66.04,11.05
  Top 0.406: U$4.A1 73.66,12.45 72.26,11.05 66.04,11.05 65.13,11.05 RN1.4
  Bottom 0.254: v63.5,24.13 63.5,13.97 64.14,13.34 65.41,13.34 v66.04,12.7
N$18  (via drill 0.5)
  Top 0.254: IC3.13 64.46,24.44 v64.77,24.13 | v64.77,14.61 64.77,12.32 64.26,11.81 64.26,10.29 64.39,10.16 65.04,10.16 RN1.3
  Top 0.406: U$4.A2 65.08,10.16 RN1.3
  Bottom 0.254: v64.77,24.13 v64.77,14.61
N$20
  Top 0.254: IC3.6 63.12,33.46 63.12,32.64 63.63,32.13 67.18,32.13 67.94,32.89 67.94,34.92 68.58,35.56 82.3,35.56 83.57,36.83 88.27,36.83 88.92,37.49 CD2.1 88.92,40.66 89.53,41.27 92.71,41.27 94.61,43.18 97.16,43.18 97.79,43.81 97.79,72.39 101.6,76.2 111.12,76.2 113.03,78.1 113.03,79.33 X11.1
N$21
  Top 1.016: ACS4.2 22.86,52.07 18.41,56.52 18.41,70.49 21.59,73.66 21.59,76.79 X7.2 24.77,77.47 24.77,73.66 22.23,71.12 22.23,53.98 23.5,52.7 24.13,52.07 ACS4.1
  Top 1.27: 23.5,52.7 23.5,56.52 22.86,57.15 22.86,53.98
N$22
  Top 1.016: ACS4.4 20.32,50.8 K5_B2.COM 21.59,49.53 ACS4.3
N$23
  Top 2.54: 133.99,79.38 133.35,79.38
N$24
  Top 0.254: IC3.8 61.86,32.37 63.12,31.12 67.82,31.12 68.96,32.26 68.96,34.29 69.22,34.54 82.8,34.54 84.07,35.81 99.95,35.81 100.33,36.2 100.33,39.09 CD1.1 100.35,71.14 102.87,73.66 126.36,73.66 128.27,75.56 128.27,79.33 X10.1
N$25
  Top 0.254: IC3.5 63.81,32.96 64.14,32.64 66.67,32.64 67.31,33.27 67.31,35.56 67.94,36.2 82.17,36.2 83.19,37.21 83.19,39.09 CD6.1 83.21,41.3 84.45,42.55 91.44,42.55 93.34,44.45 95.89,44.45 96.52,45.09 96.52,72.98 X11.3 102.87,79.33 102.87,79.38
N$31  (via drill 0.5)
  Top 1.016: C2.2 C4.2 87.55,24.36 U$5.IN 90.81,24.1 v90.81,25.4 | BRA3.+ v88.9,10.16
  Bottom 1.016: v88.9,10.16 90.17,10.16 90.81,10.79 v90.81,25.4
N$33
  Top 0.254: CE1.1 74.91,41.81 ACS1.6
N$34
  Top 0.254: CE2.1 57.13,41.81 ACS2.6
N$35
  Top 0.254: CE3.1 39.35,41.81 ACS3.6
N$36
  Top 0.254: CE4.1 21.57,41.81 ACS4.6
N$42
  Top 1.016: ACS1.3 74.93,49.53 K8_B2.COM 73.66,50.8 ACS1.4
N$43
  Top 1.016: K8_B2.NC 67.06,70.1 64.14,73.03 64.14,78.69 X4.3
N$44
  Top 1.016: K8_B2.NO 78.99,70.87 74.3,75.56 74.3,78.69 X4.1
N$45
  Top 1.016: K7_B2.NO 61.21,69.6 59.05,71.75 59.05,78.69 X5.1
N$46
  Top 1.016: K6_B2.NO 43.43,78.31 X6.1
N$47  (via drill 0.5)
  Top 0.254: RN2.2 101.96,21.57 101.73,21.34 101.73,20.07 101.35,19.69 v100.33,19.69
  Top 0.406: IC4.5 104.01,21.08 103.5,21.59 102.55,21.59 RN2.2
  Bottom 0.254: v100.33,19.69 100.97,19.05 100.97,14.99 100.33,14.35 U$18.B1
N$48  (via drill 0.5)
  Top 0.254: v100.97,24.77 101.73,24 101.73,22.61 101.98,22.35 102.51,22.35 RN2.3
  Top 0.406: IC4.4 102.55,22.35 RN2.3
  Bottom 0.406: U$18.B2 101.35,11.81 101.6,12.07 101.6,23.5 100.97,24.13 v100.97,24.77
N$49  (via drill 0.5)
  Top 0.406: IC4.3 102.98,23.62 RN2.4 102.49,23.21 v102.49,24.77
  Bottom 0.406: U$18.B3 102.23,9.27 102.49,9.53 v102.49,24.77
N$50
  Top 0.305: RN5.7 112.5,17.89 113.03,18.41 115.15,18.41 IC4.12 116.91,18.48 118.11,19.69 120.45,19.69 IC5.6
N$51
  Top 0.305: RN5.6 113.3,16.78 113.67,17.14 115.15,17.14 IC4.11 116.91,17.21 118.11,18.41 120.45,18.41 IC5.7
N$52
  Top 0.254: 115.15,15.88 IC4.10
  Top 0.305: RN5.5 114.1,14.83 IC4.10 116.91,15.94 118.11,17.14 120.45,17.14 IC5.8
N$53
  Top 0.406: RN3.1 136.06,13.5 135.25,12.7 120.4,12.7 119.89,12.19 119.89,9.54 R1.C
N$54
  Top 0.406: RN3.2 136.93,18.65 137.16,18.41 137.16,13.34 135.89,12.07 125.98,12.07 125.6,11.68 125.6,9.54 R2.C
N$55
  Top 0.406: RN3.3 137.4,19.45 137.79,19.05 137.79,12.7 136.53,11.43 131.95,11.43 131.32,10.79 131.32,9.54 R3.C
N$56
  Top 0.406: RN3.4 137.87,20.25 138.43,19.69 138.43,11.56 137.03,10.16 137.03,9.54 R4.C
N$89
  Top 0.305: RN5.8 111.7,18.99 112.39,19.69 115.15,19.69 IC4.13 116.91,19.75 118.11,20.96 120.45,20.96 IC5.5
N$97
  Bottom 2.54: 128.27,79.33 128.29,79.35
N$103
  Bottom 2.54: 138.43,79.33 138.45,79.35
N$137
  Top 1.016: K7_B2.NC 49.28,78.35 X5.3
N$138
  Top 1.016: ACS2.4 55.88,50.8 K7_B2.COM 56.52,50.16 | ACS2.3 57.15,49.53 56.52,50.16 | 56.52,50.16 56.52,46.99
N$139
  Top 1.016: K6_B2.NC 31.5,70.23 33.66,72.39 33.66,78.69 X6.3
N$140
  Top 1.016: ACS3.4 38.1,50.8 K6_B2.COM 39.37,49.53 ACS3.3
N$141
  Top 1.016: K5_B2.NC 13.72,70.87 18.41,75.56 18.41,78.69 X7.3
N$143
  Top 1.016: K5_B2.NO 25.65,70.1 28.57,73.03 28.57,78.69 X7.1
N$162
  Top 1.016: 20.95,49.53 20.95,46.99
N$163
  Top 1.016: 23.5,52.07 23.5,46.99
N$164
  Top 1.016: 21.59,53.98 21.59,71.75 24.13,74.29 24.13,76.84 23.5,77.47 22.86,76.84 | 22.86,76.84 22.23,76.2 22.23,73.66 23.5,74.93 23.5,76.2 22.86,76.84 | 22.86,76.84 22.86,73.66 19.05,69.85 19.05,57.15 20.95,55.24 20.95,55.88 20.95,70.49 | 20.95,71.12 20.95,70.49 | 20.95,70.49 19.68,69.22 19.68,57.79 20.32,57.15 20.32,69.22
  Top 1.27: 20.95,54.61 20.95,55.88
N$165
  Top 1.016: 38.73,49.53 38.73,46.99
N$166
  Top 1.016: 41.27,52.07 41.27,46.99 | ACS3.2 40.64,52.07 36.2,56.52 36.2,70.49 36.83,71.12 36.83,76.79 X6.2 40.01,77.47 40.01,55.24 40.01,53.98 41.91,52.07 ACS3.1
  Top 1.27: 41.27,52.07 41.27,53.98 | 41.27,53.98 40.01,55.24 | 39.37,54.61 40.01,53.98 | 41.27,53.98 41.27,56.52 40.64,57.15 40.64,55.24
N$167
  Top 1.016: 39.37,53.98 37.47,55.88 | 37.47,55.88 36.83,56.52 36.83,69.85 38.1,71.12 38.1,78.1 38.73,78.74 38.73,70.49 | 38.73,70.49 38.73,55.88 39.37,55.24 39.37,77.47 | 37.47,76.84 37.47,55.88 | 37.47,55.88 38.1,56.52 38.1,69.85 38.73,70.49
N$168
  Top 1.016: 59.05,52.07 59.05,46.99
N$170
  Top 1.016: 56.52,67.94 55.88,67.94 53.98,69.85 53.98,76.84 54.61,76.84 | 57.15,53.98 53.34,57.79 53.34,76.84 53.98,77.47 54.61,76.84 | 54.61,76.84 55.24,76.2 55.24,56.52 55.88,55.88 | 55.88,55.88 57.15,54.61 57.15,67.94 55.88,69.22 55.88,55.88 | 55.88,55.88 56.52,56.52 56.52,67.31 | 54.61,76.84 54.61,57.79 | 54.61,57.15 54.61,57.79 | 54.61,57.79 53.98,58.42 53.98,69.22
N$171
  Top 1.016: 74.3,49.53 74.3,46.99
N$172
  Top 1.016: 76.83,52.07 76.83,46.99
N$173
  Top 1.016: 70.48,74.29 70.48,76.84 69.22,78.1 68.58,77.47 67.94,77.47 67.94,75.56 71.12,72.39 71.12,57.79 74.93,53.98 74.93,54.61 | 70.48,74.29 70.48,73.66 74.93,69.22 74.93,55.24 | 70.48,74.29 68.58,76.2 68.58,76.84 69.22,77.47 69.85,76.84 69.85,76.2 | 69.85,75.56 69.85,76.2 | 69.85,76.2 69.22,76.84
N$174
  Top 1.016: 74.3,55.24 74.3,69.22 71.75,71.75 71.75,57.79 72.39,57.15 | 73.03,56.52 73.66,55.88 73.66,69.22 72.39,70.49 72.39,57.15 | 72.39,57.15 73.03,56.52 | 73.03,56.52 73.03,69.22
N$305
  Top 2.54: 64.16,78.72 64.16,73 66.67,70.49 66.67,66.04 67.06,65.66
N$306
  Top 2.54: 74.32,78.72 74.32,75.54 78.74,71.12 78.74,65.91 78.99,65.66
N$307
  Top 2.54: 59.08,78.72 59.08,71.73 60.96,69.85 60.96,65.91 61.21,65.66
N$308
  Top 2.54: 43.84,78.72 43.84,66.06 43.43,65.66
N$309
  Top 2.54: 48.92,78.72 48.92,66.02 49.28,65.66
N$311
  Top 2.54: 33.68,78.72 33.68,71.78 31.75,69.85 31.75,65.91 31.5,65.66
N$313
  Top 2.54: 18.44,78.72 18.44,74.95 13.34,69.85 13.34,66.04 13.72,65.66
N$315
  Top 2.54: 28.6,78.72 28.6,73.05 25.4,69.85 25.4,65.91 25.65,65.66
N$360
  Top 2.54: 28.6,78.72 28.6,73.05 26.04,70.49 26.04,66.04 25.65,65.66
N$361
  Top 2.54: 18.44,78.72 18.44,74.95 13.97,70.49 13.97,65.91 13.72,65.66
N$363
  Top 2.54: 43.84,78.72 43.84,66.06 43.43,65.66
N$364
  Top 2.54: 33.68,78.72 33.68,71.78 31.75,69.85 31.75,65.91 31.5,65.66
N$366
  Top 2.54: 59.08,78.72 59.08,71.1 60.96,69.22 60.96,65.91 61.21,65.66
N$367
  Top 2.54: 48.92,78.72 48.92,66.02 49.28,65.66
N$369
  Top 2.54: 74.32,78.72 74.32,75.54 78.74,71.12 78.74,65.91 78.99,65.66
N$370
  Top 2.54: 64.16,78.72 64.16,73.64 67.31,70.49 67.31,65.91 67.06,65.66
N$373
  Bottom 2.54: 13.72,65.66 13.72,70.23 18.41,74.93 18.41,78.69 18.44,78.72
N$374
  Bottom 2.54: 25.65,65.66 25.65,69.47 28.57,72.39 28.57,78.69 28.6,78.72
N$375
  Bottom 2.54: 43.43,65.66 43.43,68.2 43.81,68.58 43.81,78.69 43.84,78.72
N$376
  Bottom 2.54: 61.21,65.66 61.21,68.96 59.05,71.12 59.05,78.69 59.08,78.72
N$377
  Bottom 2.54: 31.5,65.66 31.5,68.96 33.66,71.12 33.66,78.69 33.68,78.72
N$379
  Bottom 2.54: 49.28,65.66 49.28,68.2 48.9,68.58 48.9,77.42 48.92,78.72
N$380
  Top 2.54: 48.9,67.94 48.9,78.74 49.53,78.74 49.53,67.94 | 48.9,67.94 49.53,67.94 | 49.53,67.94 49.53,67.31 | 49.53,67.31 49.53,65.41 48.9,65.41 48.9,66.04 | 48.9,66.04 48.9,67.31 | 48.9,67.94 48.9,67.31 | 48.9,67.31 49.53,67.31 | 48.9,66.04 50.16,66.04 | 50.16,66.04 50.16,78.74 47.62,78.74 47.62,64.77 50.16,64.77 50.16,66.04
N$383
  Top 2.54: 58.42,78.74 58.42,71.12 60.33,69.22 60.33,64.77 62.23,64.77 62.23,69.85 59.69,72.39 59.69,78.74 58.42,78.74
N$384
  Top 2.54: 66.04,64.77 66.04,70.49 63.5,73.03 63.5,78.74 64.77,78.74 64.77,73.66 67.94,70.49 67.94,64.77 66.04,64.77
N$386
  Top 2.54: 73.66,78.74 73.66,75.56 78.11,71.12 78.11,64.77 80.01,64.77 80.01,71.12 74.93,76.2 74.93,78.74 73.66,78.74
N$387
  Top 2.54: 44.45,78.74 44.45,64.77 42.55,64.77 42.55,78.74 44.45,78.74
N$389
  Top 2.54: 34.29,78.74 34.29,71.75 33.02,70.49 33.02,64.77 30.48,64.77 30.48,69.85 33.02,72.39 33.02,78.74 34.29,78.74
N$390
  Top 2.54: 28.57,78.74 29.21,78.74 29.21,73.03 26.67,70.49 26.67,64.77 24.77,64.77 24.77,69.85 27.94,73.03 | 28.57,73.66 28.57,78.74 | 28.57,78.74 27.94,78.74 27.94,72.39
N$392
  Top 2.54: 19.05,78.74 19.05,74.93 14.61,70.49 14.61,64.77 12.7,64.77 12.7,69.85 17.78,74.93 17.78,78.74 19.05,78.74
N$393
  Bottom 2.54: 18.41,78.74 17.78,78.74 17.78,74.93 12.7,69.85 12.7,64.77 14.61,64.77 14.61,70.49 19.05,74.93 19.05,78.74
N$395
  Bottom 2.54: 27.94,78.74 27.94,73.03 24.77,69.85 24.77,64.77 26.67,64.77 26.67,70.49 29.21,73.03 29.21,78.74 27.94,78.74
N$396
  Bottom 2.54: 33.02,78.74 33.02,72.39 30.48,69.85 30.48,64.77 33.02,64.77 33.02,70.49 34.29,71.75 34.29,78.74 33.02,78.74
N$398
  Bottom 2.54: 44.45,78.74 42.55,78.74 42.55,64.77 44.45,64.77 44.45,78.74
N$399
  Bottom 2.54: 47.62,78.74 47.62,64.77 50.16,64.77 50.16,78.74 47.62,78.74
N$401
  Bottom 2.54: 58.42,78.74 58.42,71.12 60.33,69.22 60.33,64.77 62.23,64.77 62.23,69.85 59.69,72.39 59.69,78.74 58.42,78.74
N$402
  Bottom 2.54: 67.06,65.66 67.06,69.47 66.04,70.49 | 66.04,70.49 64.14,72.39 | 64.14,72.39 64.14,78.69 64.16,78.72 | 64.14,72.39 63.5,73.03 63.5,78.74 64.77,78.74 64.77,73.66 67.94,70.49 67.94,64.77 66.04,64.77 66.04,70.49
N$404
  Bottom 2.54: 78.99,65.66 78.99,70.23 78.11,71.12 | 78.11,71.12 74.3,74.93 | 74.3,74.93 74.3,78.69 74.32,78.72 | 74.3,74.93 73.66,75.56 73.66,78.74 74.93,78.74 74.93,76.2 80.01,71.12 80.01,64.77 78.11,64.77 78.11,71.12
OC_R1  (via drill 0.5)
  Top 0.305: IC5.11 132.59,17.27 133.22,17.91 134.4,17.91 RN3.8
  Top 0.406: v128.27,17.14 130.25,17.14 IC5.11
  Bottom 0.406: K8_B2.C1 78.99,37.85 80.01,36.83 121.28,36.83 122.56,35.56 122.56,17.78 123.19,17.14 v128.27,17.14
OC_R2  (via drill 0.5)
  Top 0.305: IC5.12 132.72,18.54 132.84,18.67 134.44,18.67 RN3.7
  Top 0.406: v128.27,18.41 130.25,18.41 IC5.12 | v121.28,34.92 v123.83,34.92
  Bottom 0.406: K7_B2.C1 62.74,51.94 62.74,36.07 63.25,35.56 120.65,35.56 v121.28,34.92 | v123.83,34.92 123.83,19.05 124.46,18.41 v128.27,18.41
OC_R3  (via drill 0.5)
  Top 0.305: IC5.13 132.59,19.81 132.97,19.43 134.44,19.43 RN3.6
  Top 0.406: v128.27,19.69 130.25,19.69 IC5.13 | v121.28,33.02 v125.09,33.02
  Bottom 0.406: 128.4,19.81 v128.27,19.69 125.73,19.69 125.09,20.32 v125.09,33.02 | K6_B2.C1 43.43,45.47 44.45,44.45 60.96,44.45 62.1,43.31 62.1,35.69 62.87,34.92 119.38,34.92 v121.28,33.02
OC_R4  (via drill 0.5)
  Top 0.305: IC5.14 132.59,21.08 133.35,20.32 134.38,20.32 RN3.5
  Top 0.406: v128.27,20.96 130.25,20.96 IC5.14 | v121.28,31.12 v126.36,31.12
  Bottom 0.406: 128.4,21.08 v128.27,20.96 127,20.96 126.36,21.59 v126.36,31.12 | K5_B2.C1 25.65,44.83 26.8,43.69 60.58,43.81 61.47,42.93 61.47,35.31 62.48,34.29 118.11,34.29 v121.28,31.12
REG_5V  (via drill 0.5, 0.9)
  Top 0.254: U$4.B2 U$4.B1 | v70.48,26.16 CA4.1 | 113.03,26.67 108.58,22.23 108.58,20.45 107.95,19.81 | IC3.16 66.41,28.31 v67.31,29.21 | v62.48,29.08 62.48,27.48 IC3.10 62.48,27.43 62.48,26.54 62.23,26.29 62.23,26.04 | RNE.6 RNE.5
  Top 0.305: H1.1 6.19,19.27 4.95,18.03 4.95,15.83 RNB.6
  Top 0.406: IC3.16 70.23,27.46 CA4.1 75.33,27.71 76.2,28.57 76.2,30.48 C1.+ | CB3.2 84.22,29.62 | IC4.18 113.54,26.16 113.03,26.67 v113.03,27.94 113.03,30.12 CB6.2 CA7.2 | 127,7.62 121.92,7.62 121.4,8.14 R1.A 121.4,11.32 v121.28,11.43 | 127,7.62 132.72,7.62 | 132.72,7.62 138.43,7.62 138.54,7.74 R4.A | R3.A 132.83,7.74 132.72,7.62 | R2.A 127.11,7.74 127,7.62 | 107.95,19.81 IC4.6 105.89,19.69 103.5,19.69 102.23,18.41 99.69,18.41 99.06,17.78 99.06,16.51 98.42,15.88 94.61,15.88 93.98,15.24 U$18.A1 U$18.A2 U$18.A3 | RNE.5 45.55,28.74 46.35,27.94 46.35,12.07
  Top 0.762: 83.82,28.57 84.45,27.94 107.95,27.94 108.58,28.57 108.58,29.82
  Top 0.813: 16.13,20.83 9.96,20.83 H1.1 | 16.13,20.83 17.27,20.83 18.41,19.69 20.75,19.69 C7.1 | IC1.4 16.13,19.15 16.13,20.83 | S1.1 57.78,3.81 58.42,4.45 58.42,22.23 62.23,26.04
  Top 1.016: C1.+ 76.83,29.84 78.11,28.57 83.82,28.57 84.45,29.21 84.45,29.87 CB3.2 CA3.2 82.55,33.02 v81.92,33.66 | 108.58,29.82 CA7.2 | 46.35,2.16 46.35,1.52 | 46.35,1.52 15.37,1.52 11.3,5.59 11.3,14.35 9.27,16.38 9.27,18.41 H1.1 | 22.05,19.69 22.23,19.69 22.86,20.32 22.86,28.57 v23.5,29.21 | S1.1 53.98,2.41 53.09,1.52 46.35,1.52
  Top 1.27: 20.75,19.69 22.05,19.69
  Top 1.778: X3.2 46.35,12.07 46.35,2.16
  Bottom 0.254: U$4.B1 76.2,13.97 75.56,14.61 71.12,14.61 70.48,15.24 v70.48,26.16 | v67.31,29.21 62.87,29.21 v62.48,29.08
  Bottom 0.406: v121.28,11.43 114.3,11.43 113.67,12.07 113.67,27.3 v113.03,27.94
  Bottom 0.61: C10.+ 76.45,24.51 74.93,26.04 74.93,29.21 C1.+
REG_5V_A  (via drill 0.5)
  Top 0.406: ACS1.8 77.47,44.45 | ACS2.8 59.69,44.45 | ACS3.8 41.91,44.45 | ACS4.8 24.13,44.45
  Top 1.016: C3.2 C5.2 87.55,16.28 U$5.OUT 89.31,19.91 v88.9,20.32 | 24.13,44.45 41.91,44.45 59.69,44.45 77.47,44.45 v87,44.45 | v106.05,44.45 106.05,36.2 v101.6,31.75
  Bottom 1.016: v87,44.45 v106.05,44.45 | v101.6,31.75 90.17,31.75 88.9,30.48 v88.9,20.32
REG_12V  (via drill 0.5)
  Top 0.61: IC1.7 13.46,23.16 | 14.1,22.48 14.15,22.48
  Top 0.813: v18.41,22.48 14.15,22.48 13.46,23.16 | v25.4,22.48 26.04,22.48 26.67,21.84 C6.1 26.67,14.61 27.94,13.34 BRA1.+
  Bottom 0.813: v18.41,22.48 v25.4,22.48
UNREG_12V  (via drill 0.5, 0.9)
  Top 0.406: v133.35,15.24 132.84,15.24 132.08,16 IC5.10
  Top 0.61: BRA3.~@1 111.12,6.99 112.39,8.26 112.39,8.89 113.03,9.53 115.57,9.53 116.2,10.16 116.2,13.97 116.84,14.61 129.54,14.61 130.18,15.24 130.18,15.8 IC5.10
  Top 1.016: BRA3.~@2 BRA3.~@1 v62.87,6.99
  Top 1.422: v31.11,33.66 15.49,33.66 13.72,35.43 K5_B2.C2
  Top 2.54: X2.2 28.87,5.42 24.13,10.16 BRA1.~@1 24.13,15.24 | 24.13,15.24 BRA1.~@2 | U$1.TIP 15.14,13.87 16.51,15.24 24.13,15.24
  Bottom 1.016: v62.87,6.99 62.87,11.43 58.42,15.88 58.42,33.02 57.78,33.66 v31.11,33.66 | 67.31,53.21 K8_B2.C2 67.06,54.86 65.41,56.52 49.53,56.52 | 49.53,56.52 31.75,56.52 | 31.75,56.52 13.97,56.52 13.72,56.26 K5_B2.C2 | K6_B2.C2 31.5,56.26 31.75,56.52 | K7_B2.C2 49.28,56.26 49.53,56.52 | v133.35,15.24 133.35,17.78 137.16,21.59 C11.+
  Bottom 1.778: v31.11,33.66 31.11,6.71 X2.2

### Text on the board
tNames: IP- | IP+ | IP- | IP- | IP+ | IP- | IP- | IP+ | IP- | IP- | IP+ | IP- | ANALOG TO DIGITAL | DIGITAL I/O | AD5 | GND | AD6 | AD7 | GND | AD8 | GP7 | GND | GP6 | GP5 | GND | GP4 | NC | COM | NO | NC | COM | NO | NC | COM | NO | NC | COM | NO | 4 | 1 | Bank 1 | REV.A | MCP23008 | 4 | 4 | 3 | 3 | 2 | 2 | 1 | 1 | 2016 ControlEverything.com | ADS7828 | SCCMR4xAD4IO4 | SC | I2C OUT | SCL | SDA | +5V | GND | A0 | A1 | A1 | A0 | A2 | ADC Address | Relay Address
